PROGRAM MAIN
VAR
	fbTest		: FB_TEST;
	{attribute 'OPC.UA.DA' := '1'}	
	fbTest2		: FB_TEST;
	
	(* Variables for input and output arguments of FB *)
	{attribute 'OPC.UA.DA' := '1'}
	value1		: INT;
	{attribute 'OPC.UA.DA' := '1'}
	value2		: INT;
	{attribute 'OPC.UA.DA' := '1'}
	nOutput1 	: INT;
	{attribute 'OPC.UA.DA' := '1'}
	nOutput2	: INT; 
END_VAR

fbTest2(
	nInput1 := value1,
	nInput2 := value2,
	nOutput1 => nOutput1,
	nOutput2 => nOutput2
);

END_PROGRAM
